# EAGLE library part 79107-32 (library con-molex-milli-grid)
RECEPTACAL
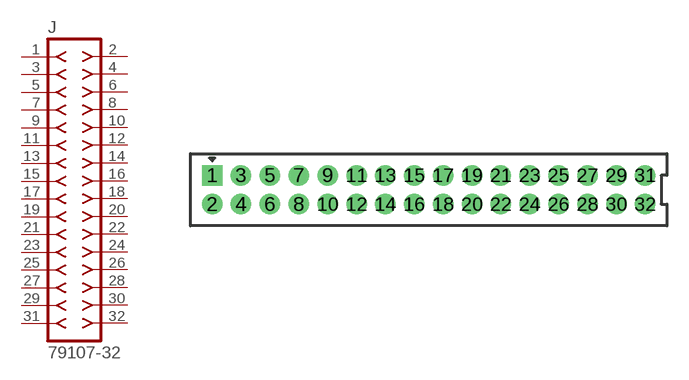
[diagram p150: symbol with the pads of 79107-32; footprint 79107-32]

Designator prefix J

## 79107-32  [79107-32]
1  1  pas
2  2  pas
3  3  pas
4  4  pas
5  5  pas
6  6  pas
7  7  pas
8  8  pas
9  9  pas
10  10  pas
11  11  pas
12  12  pas
13  13  pas
14  14  pas
15  15  pas
16  16  pas
17  17  pas
18  18  pas
19  19  pas
20  20  pas
21  21  pas
22  22  pas
23  23  pas
24  24  pas
25  25  pas
26  26  pas
27  27  pas
28  28  pas
29  29  pas
30  30  pas
31  31  pas
32  32  pas

## Footprint 79107-32 (pad centres in mm)
RECEPTACAL Dual Row, Vertical, Through-Hole
drill 0.914 square: 1 -15,1
drill 0.914: 2 -15,-1; 3 -13,1; 4 -13,-1; 5 -11,1; 6 -11,-1; 7 -9,1; 8 -9,-1; 9 -7,1; 10 -7,-1; 11 -5,1; 12 -5,-1; 13 -3,1; 14 -3,-1; 15 -1,1; 16 -1,-1; 17 1,1; 18 1,-1; 19 3,1; 20 3,-1; 21 5,1; 22 5,-1; 23 7,1; 24 7,-1; 25 9,1; 26 9,-1; 27 11,1; 28 11,-1; 29 13,1; 30 13,-1; 31 15,1; 32 15,-1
